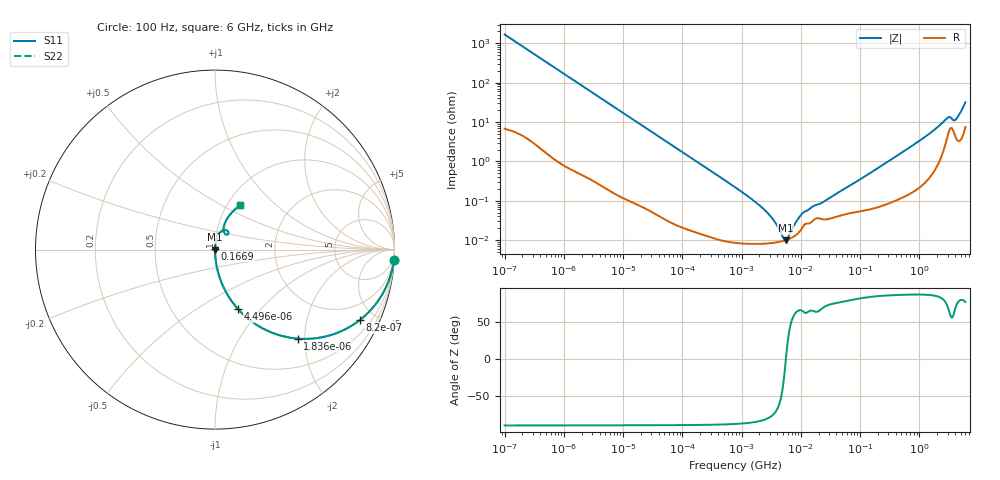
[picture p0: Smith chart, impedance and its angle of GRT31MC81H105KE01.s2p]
!Murata Part Number: GRT31MC81H105KE01
!These Parameters are Measured in Series Mode Connection
!Data Generated on Jun 19, 2026
!  o--ll--o
!Port1  Port2
!  o------o
!Operation Temp=25[degC], DC Bias Voltage=0[V]
!Freq. Start=100[Hz] Stop=6[GHz] 401[Steps]
# Hz S RI R 50
!Freq.(Hz) S11(Real) S11(Imag) S21(Real) S21(Imag) S12(Real) S12(Imag) S22(Real) S22(Imag)
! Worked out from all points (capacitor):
!   401 points, 100 Hz to 6 GHz, reference 50 ohm
!   read as one part in series: C = 947 nF near 109 Hz
!   lowest |Z| = 9.95 mohm at 5.555 MHz (marker M1)
!   series resonance near 5.604 MHz, so ESL is about 850 pH
!   S11 on the Smith chart (normalised r, x): 100 Hz: 1, -34; 820 Hz: 1.02, -4.12; 1.836 kHz: 1.01, -1.85; 4.496 kHz: 1.00, -0.76; 166.9 MHz: 1.00, +0.01; 6 GHz: 1.15, +0.62
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100  0.9962 -0.0593  0.00377 0.0593  0.00377 0.0593  0.9962 -0.0593
383  0.95 -0.2153  0.05 0.2153  0.05 0.2153  0.95 -0.2153
820  0.8086 -0.3912  0.1914 0.3912  0.1914 0.3912  0.8086 -0.3912
1836  0.4603 -0.4958  0.5397 0.4958  0.5397 0.4958  0.4603 -0.4958
2008  0.4166 -0.4903  0.5834 0.4903  0.5834 0.4903  0.4166 -0.4903
4496  0.1267 -0.3296  0.8733 0.3296  0.8733 0.3296  0.1267 -0.3296
12041  0.0207 -0.1387  0.9793 0.1387  0.9793 0.1387  0.0207 -0.1387
40335  0.00221 -0.0425  0.9978 0.0425  0.9978 0.0425  0.00221 -0.0425
774597  8.97e-05 -0.00221  0.9999 0.00221  0.9999 0.00221  8.97e-05 -0.00221
2594782  8.18e-05 -0.000528  0.9999 0.000528  0.9999 0.000528  8.18e-05 -0.000528
3549919  8.56e-05 -0.000295  0.9999 0.000295  0.9999 0.000295  8.56e-05 -0.000295
5079039  9.54e-05 -6.14e-05  0.9999 6.14e-05  0.9999 6.14e-05  9.54e-05 -6.14e-05
5554849  9.93e-05 -5.4e-06  0.9999 5.4e-06  0.9999 5.4e-06  9.93e-05 -5.4e-06
6075234  0.000104 5.08e-05  0.9999 -5.08e-05  0.9999 -5.08e-05  0.000104 5.08e-05
9941735  0.000178 0.000385  0.9998 -0.000385  0.9998 -0.000385  0.000178 0.000385
1.555665e7  0.0003 0.000629  0.9997 -0.000629  0.9997 -0.000629  0.0003 0.000629
1.669249e8  0.000664 0.00563  0.9993 -0.00563  0.9993 -0.00563  0.000664 0.00563
3.124326e8  0.000969 0.0104  0.999 -0.0104  0.999 -0.0104  0.000969 0.0104
1.309207e9  0.00499 0.0437  0.995 -0.0437  0.995 -0.0437  0.00499 0.0437
2.931063e9  0.0487 0.1083  0.9513 -0.1083  0.9513 -0.1083  0.0487 0.1083
4.009986e9  0.0519 0.0925  0.9481 -0.0925  0.9481 -0.0925  0.0519 0.0925
6e9  0.1404 0.2467  0.8596 -0.2467  0.8596 -0.2467  0.1404 0.2467
